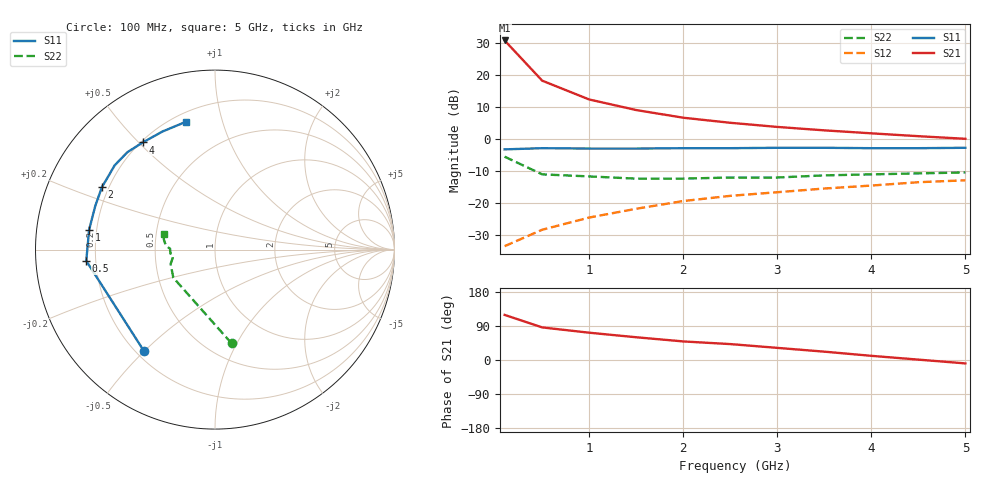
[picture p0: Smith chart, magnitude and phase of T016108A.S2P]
!AT-01610
!S-PARAMETERS at Vce=8V  Ic=35mA.  LAST UPDATED 07-21-92
!OBSOLETED Feb 1994 - nearest replacement: AT-42010
# ghz s ma r 50
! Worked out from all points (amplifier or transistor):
!   11 points, 100 MHz to 5 GHz, reference 50 ohm
!   highest |S21| = 30.9 dB at 100 MHz (marker M1)
!   |S21| within 3 dB of that: start of sweep to 195.2 MHz
!   unconditionally stable (mu >= 1): 727.5 MHz to end of sweep
!   at 500 MHz: K = 0.87, MSG = 23.4 dB, |S12| = -28.4 dB
!   at 2.5 GHz: K = 1.18, MAG = 8.9 dB, |S12| = -17.8 dB
!   at 5 GHz: K = 1.11, MAG = 4.5 dB, |S12| = -12.9 dB
!   S11 on the Smith chart (normalised r, x): 100 MHz: 0.23, -0.50; 500 MHz: 0.16, -0.04; 1 GHz: 0.17, +0.08; 2 GHz: 0.17, +0.25; 4 GHz: 0.21, +0.51; 5 GHz: 0.25, +0.76
0.1  0.69 -125.0  35.08 119.0  0.021 44.0  0.53 -80.0
0.5  0.72 -175.0  8.22 86.0  0.038 45.0  0.28 -146.0
1  0.71 171.0  4.17 72.0  0.059 50.0  0.26 -162.0
1.5  0.71 160.0  2.85 60.0  0.081 56.0  0.24 -169.0
2  0.72 151.0  2.16 49.0  0.107 50.0  0.24 -174.0
2.5  0.72 147.0  1.8 42.0  0.129 51.0  0.25 -175.0
3  0.73 140.0  1.55 32.0  0.147 47.0  0.25 179.0
3.5  0.73 132.0  1.37 22.0  0.168 41.0  0.27 176.0
4  0.72 124.0  1.23 11.0  0.187 36.0  0.28 173.0
4.5  0.72 114.0  1.11 1.0  0.211 30.0  0.29 169.0
5  0.73 103.0  1.01 -9.0  0.226 23.0  0.3 163.0
